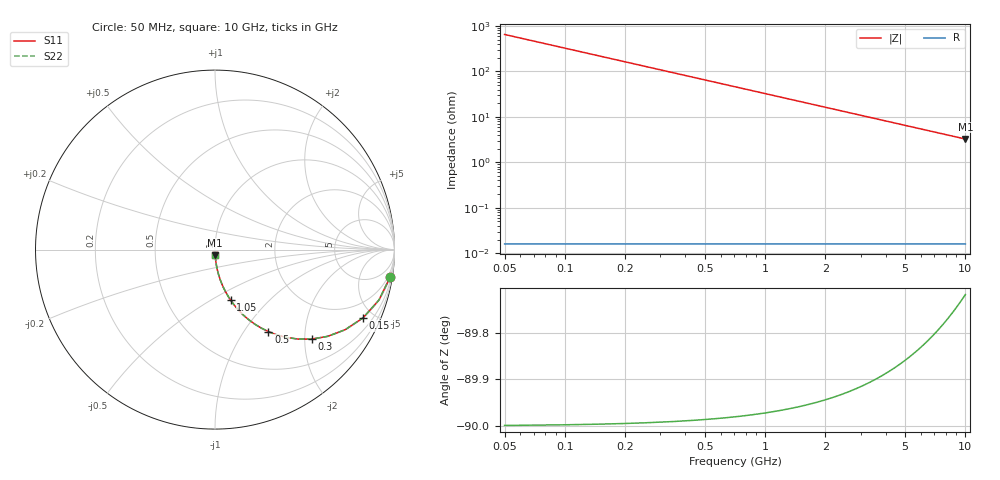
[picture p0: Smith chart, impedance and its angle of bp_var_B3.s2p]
! Created Fri Sep 21 13:02:36 2018
# hz S ma R 50
! 2 Port Network Data from SP1.SP block
! freq  magS11  angS11  magS21  angS21  magS12  angS12  magS22  angS22
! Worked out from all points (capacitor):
!   200 points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, 50 MHz to 10 GHz, reference 50 ohm
!   read as one part in series: C = 4.89 pF near 100 MHz
!   lowest |Z| = 3.25 ohm at 10 GHz (marker M1)
!   S11 on the Smith chart (normalised r, x): 50 MHz: 1, -13; 150 MHz: 1.00, -4.34; 300 MHz: 1.00, -2.17; 500 MHz: 1.00, -1.30; 1.05 GHz: 1.00, -0.62; 10 GHz: 1.00, -0.07
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5e7  0.9884 -8.7  0.1519 81.3  0.1519 81.3  0.9884 -8.7
1e8  0.9558 -17.1  0.2938 72.9  0.2938 72.9  0.9558 -17.1
1.5e8  0.9081 -24.8  0.4187 65.2  0.4187 65.2  0.9081 -24.8
2e8  0.8518 -31.6  0.5237 58.4  0.5237 58.4  0.8518 -31.6
2.5e8  0.7928 -37.5  0.6093 52.5  0.6093 52.5  0.7928 -37.5
3e8  0.735 -42.7  0.6779 47.3  0.6779 47.3  0.735 -42.7
4e8  0.6309 -50.9  0.7758 39.1  0.7758 39.1  0.6309 -50.9
5e8  0.5453 -56.9  0.8381 33.0  0.8381 33.0  0.5453 -56.9
6e8  0.4765 -61.5  0.879 28.5  0.879 28.5  0.4765 -61.5
7.5e8  0.3978 -66.5  0.9173 23.4  0.9173 23.4  0.3978 -66.5
9e8  0.3399 -70.1  0.9403 19.9  0.9403 19.9  0.3399 -70.1
1.05e9  0.2959 -72.8  0.9551 17.2  0.9551 17.2  0.2959 -72.8
1.4e9  0.2263 -76.9  0.9739 13.1  0.9739 13.1  0.2263 -76.9
1.75e9  0.1827 -79.4  0.983 10.5  0.983 10.5  0.1827 -79.4
2.1e9  0.153 -81.1  0.9881 8.8  0.9881 8.8  0.153 -81.1
2.5e9  0.129 -82.5  0.9915 7.4  0.9915 7.4  0.129 -82.5
3.4e9  0.09522 -84.4  0.9953 5.5  0.9953 5.5  0.09522 -84.4
4.15e9  0.07813 -85.4  0.9968 4.5  0.9968 4.5  0.07813 -85.4
5.05e9  0.06427 -86.2  0.9978 3.7  0.9978 3.7  0.06427 -86.2
6.7e9  0.04849 -87.0  0.9987 2.8  0.9987 2.8  0.04849 -87.0
8.35e9  0.03892 -87.5  0.9991 2.2  0.9991 2.2  0.03892 -87.5
1e10  0.03251 -87.9  0.9993 1.9  0.9993 1.9  0.03251 -87.9
